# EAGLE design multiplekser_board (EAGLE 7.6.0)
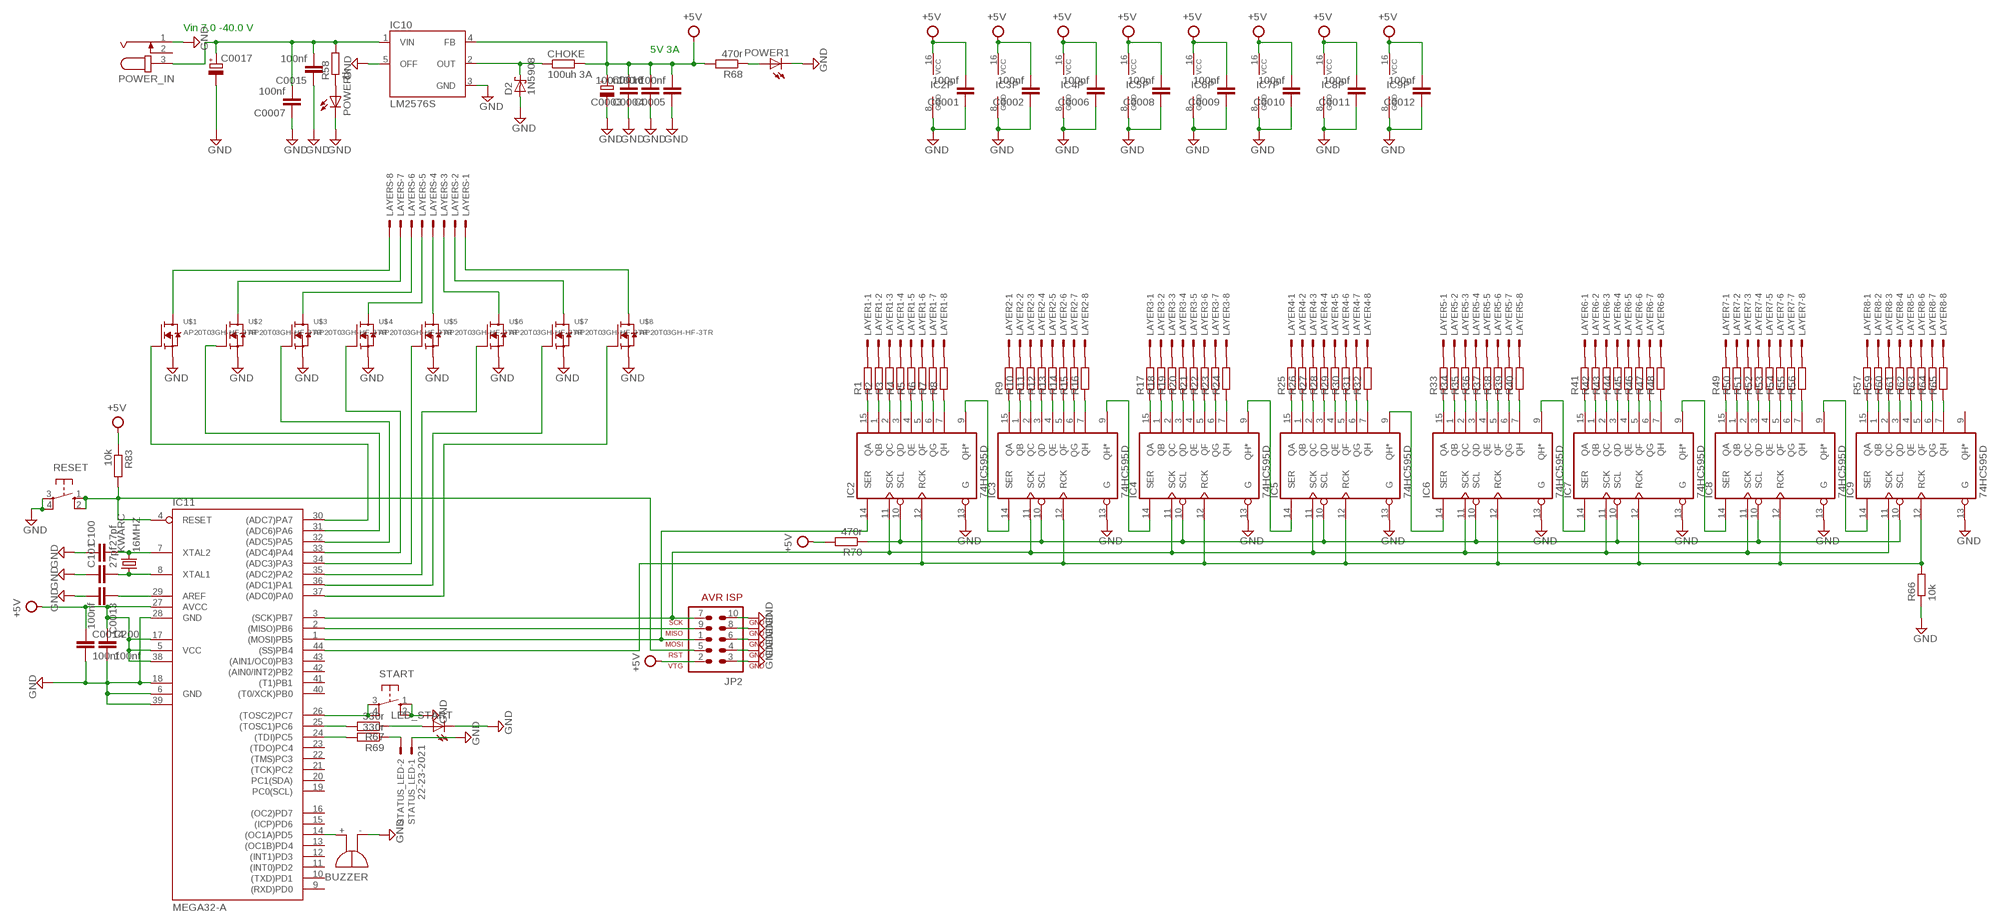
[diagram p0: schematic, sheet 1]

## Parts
BUZZER  F/QMBIII  [F/QMBIII]
C0001  100nf  C-EUC1206  [C1206]
C0002  100nf  C-EUC1206  [C1206]
C0003  100nf  C-EUC1206  [C1206]
C0004  100nf  C-EUC1206  [C1206]
C0005  100nf  C-EUC1206  [C1206]
C0006  100nf  C-EUC1206  [C1206]
C0007  100nf  C-EUC1206  [C1206]
C0008  100nf  C-EUC1206  [C1206]
C0009  100nf  C-EUC1206  [C1206]
C0010  100nf  C-EUC1206  [C1206]
C0011  100nf  C-EUC1206  [C1206]
C0012  100nf  C-EUC1206  [C1206]
C0013  100nf  C-EUC1206  [C1206]
C0014  100nf  C-EUC1206  [C1206]
C0015  100nf  C-EUC1206  [C1206]
C0016  CPOL-EUE10-30  [EB30D]
C0017  CPOL-EUE2.5-6  [E2,5-6]
C100  27pf  C-EUC1206  [C1206]
C101  27pf  C-EUC1206  [C1206]
C200  100nf  C-EUC1206  [C1206]
CHOKE  100uh 3A  R-EU_0207/12  [0207/12]
D2  1N5908  [C4111-15]
IC2  74HC595D  [SO16]
IC3  74HC595D  [SO16]
IC4  74HC595D  [SO16]
IC5  74HC595D  [SO16]
IC6  74HC595D  [SO16]
IC7  74HC595D  [SO16]
IC8  74HC595D  [SO16]
IC9  74HC595D  [SO16]
IC10  LM2576S  [TO263-5]
IC11  MEGA32-A  [TQFP44]
JP2  AVR-ISP-10ML  [ML10]
KWARC  16MHZ  CRYSTALHC49UV  [HC49U-V]
LAYER1  22-23-2081  [22-23-2081]
LAYER2  22-23-2081  [22-23-2081]
LAYER3  22-23-2081  [22-23-2081]
LAYER4  22-23-2081  [22-23-2081]
LAYER5  22-23-2081  [22-23-2081]
LAYER6  22-23-2081  [22-23-2081]
LAYER7  22-23-2081  [22-23-2081]
LAYER8  22-23-2081  [22-23-2081]
LAYERS  22-23-2081  [22-23-2081]
LED_START  LEDCHIPLED_1206  [CHIPLED_1206]
POWER  LEDCHIPLED_1206  [CHIPLED_1206]
POWER1  LEDCHIPLED_1206  [CHIPLED_1206]
POWER_IN  JACK-PLUG1  [SPC4078]
R1  R-EU_M1206  [M1206]
R2  R-EU_M1206  [M1206]
R3  R-EU_M1206  [M1206]
R4  R-EU_M1206  [M1206]
R5  R-EU_M1206  [M1206]
R6  R-EU_M1206  [M1206]
R7  R-EU_M1206  [M1206]
R8  R-EU_M1206  [M1206]
R9  R-EU_M1206  [M1206]
R10  R-EU_M1206  [M1206]
R11  R-EU_M1206  [M1206]
R12  R-EU_M1206  [M1206]
R13  R-EU_M1206  [M1206]
R14  R-EU_M1206  [M1206]
R15  R-EU_M1206  [M1206]
R16  R-EU_M1206  [M1206]
R17  R-EU_M1206  [M1206]
R18  R-EU_M1206  [M1206]
R19  R-EU_M1206  [M1206]
R20  R-EU_M1206  [M1206]
R21  R-EU_M1206  [M1206]
R22  R-EU_M1206  [M1206]
R23  R-EU_M1206  [M1206]
R24  R-EU_M1206  [M1206]
R25  R-EU_M1206  [M1206]
R26  R-EU_M1206  [M1206]
R27  R-EU_M1206  [M1206]
R28  R-EU_M1206  [M1206]
R29  R-EU_M1206  [M1206]
R30  R-EU_M1206  [M1206]
R31  R-EU_M1206  [M1206]
R32  R-EU_M1206  [M1206]
R33  R-EU_M1206  [M1206]
R34  R-EU_M1206  [M1206]
R35  R-EU_M1206  [M1206]
R36  R-EU_M1206  [M1206]
R37  R-EU_M1206  [M1206]
R38  R-EU_M1206  [M1206]
R39  R-EU_M1206  [M1206]
R40  R-EU_M1206  [M1206]
R41  R-EU_M1206  [M1206]
R42  R-EU_M1206  [M1206]
R43  R-EU_M1206  [M1206]
R44  R-EU_M1206  [M1206]
R45  R-EU_M1206  [M1206]
R46  R-EU_M1206  [M1206]
R47  R-EU_M1206  [M1206]
R48  R-EU_M1206  [M1206]
R49  R-EU_M1206  [M1206]
R50  R-EU_M1206  [M1206]
R51  R-EU_M1206  [M1206]
R52  R-EU_M1206  [M1206]
R53  R-EU_M1206  [M1206]
R54  R-EU_M1206  [M1206]
R55  R-EU_M1206  [M1206]
R56  R-EU_M1206  [M1206]
R57  R-EU_M1206  [M1206]
R58  1k  R-EU_R1206  [R1206]
R59  R-EU_M1206  [M1206]
R60  R-EU_M1206  [M1206]
R61  R-EU_M1206  [M1206]
R62  R-EU_M1206  [M1206]
R63  R-EU_M1206  [M1206]
R64  R-EU_M1206  [M1206]
R65  R-EU_M1206  [M1206]
R66  10k  R-EU_M1206  [M1206]
R67  330r  R-EU_M1206  [M1206]
R68  470r  R-EU_R1206  [R1206]
R69  330r  R-EU_M1206  [M1206]
R70  470r  R-EU_M1206  [M1206]
R83  10k  R-EU_R1206  [R1206]
RESET  10-XX  [B3F-10XX]
START  10-XX  [B3F-10XX]
STATUS_LED  22-23-2021  [22-23-2021]
U$1  AP20T03GH-HF-3TR  [TO-252]
U$2  AP20T03GH-HF-3TR  [TO-252]
U$3  AP20T03GH-HF-3TR  [TO-252]
U$4  AP20T03GH-HF-3TR  [TO-252]
U$5  AP20T03GH-HF-3TR  [TO-252]
U$6  AP20T03GH-HF-3TR  [TO-252]
U$7  AP20T03GH-HF-3TR  [TO-252]
U$8  AP20T03GH-HF-3TR  [TO-252]

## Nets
+5V: C0001.2 C0002.2 C0003.2 C0004.2 C0005.2 C0006.2 C0008.2 C0009.2 C0010.2 C0011.2 C0012.2 C0014.1 C0016.+ C200.1 CHOKE.2 IC2.16(VCC) IC3.16(VCC) IC4.16(VCC) IC5.16(VCC) IC6.16(VCC) IC7.16(VCC) IC8.16(VCC) IC9.16(VCC) IC10.4(FB) IC11.5(VCC) IC11.17(VCC1) IC11.27(AVCC) IC11.38(VCC2) JP2.2 R68.2 R70.2 R83.1
GND: BUZZER.-(+) C0001.1 C0002.1 C0003.1 C0004.1 C0005.1 C0006.1 C0007.1 C0008.1 C0009.1 C0010.1 C0011.1 C0012.1 C0013.2 C0014.2 C0015.1 C0016.- C0017.- C100.1 C101.1 C200.2 D2.A IC2.8(GND) IC2.13(G) IC3.8(GND) IC3.13(G) IC4.8(GND) IC4.13(G) IC5.8(GND) IC5.13(G) IC6.8(GND) IC6.13(G) IC7.8(GND) IC7.13(G) IC8.8(GND) IC8.13(G) IC9.8(GND) IC9.13(G) IC10.3(GND) IC10.5(OFF) IC11.6(GND) IC11.18(GND1) IC11.28(GND) IC11.39(GND2) JP2.3 JP2.4 JP2.6 JP2.8 JP2.10 LED_START.C POWER1.C POWER.C POWER_IN.1 R66.1 RESET.3(P) RESET.4(P1) START.1(S) START.2(S1) STATUS_LED.1 U$1.3(S) U$2.3(S) U$3.3(S) U$4.3(S) U$5.3(S) U$6.3(S) U$7.3(S) U$8.3(S)
N$1: IC2.15(QA) R1.1
N$2: IC2.1(QB) R2.1
N$3: IC2.2(QC) R3.1
N$4: IC2.3(QD) R4.1
N$5: IC2.4(QE) R5.1
N$6: IC2.5(QF) R6.1
N$7: IC2.6(QG) R7.1
N$8: IC2.7(QH) R8.1
N$9: IC2.9(QH*) IC3.14(SER)
N$10: IC2.11(SCK) IC3.11(SCK) IC4.11(SCK) IC5.11(SCK) IC6.11(SCK) IC7.11(SCK) IC8.11(SCK) IC9.11(SCK) IC11.3((SCK)PB7) JP2.7
N$11: IC2.12(RCK) IC3.12(RCK) IC4.12(RCK) IC5.12(RCK) IC6.12(RCK) IC7.12(RCK) IC8.12(RCK) IC9.12(RCK) IC11.44((SS)PB4) R66.2
N$12: IC3.15(QA) R9.1
N$13: IC3.1(QB) R10.1
N$14: IC3.2(QC) R11.1
N$15: IC3.3(QD) R12.1
N$16: IC3.4(QE) R13.1
N$17: IC3.5(QF) R14.1
N$18: IC3.6(QG) R15.1
N$19: IC3.7(QH) R16.1
N$20: IC4.15(QA) R17.1
N$21: IC4.1(QB) R18.1
N$22: IC4.2(QC) R19.1
N$23: IC4.3(QD) R20.1
N$24: IC4.4(QE) R21.1
N$25: IC4.5(QF) R22.1
N$26: IC4.6(QG) R23.1
N$27: IC4.7(QH) R24.1
N$28: IC4.9(QH*) IC5.14(SER)
N$29: IC5.15(QA) R25.1
N$30: IC5.1(QB) R26.1
N$31: IC5.2(QC) R27.1
N$32: IC5.3(QD) R28.1
N$33: IC5.4(QE) R29.1
N$34: IC5.5(QF) R30.1
N$35: IC5.6(QG) R31.1
N$36: IC5.7(QH) R32.1
N$37: IC3.9(QH*) IC4.14(SER)
N$38: IC6.3(QD) R36.1
N$39: IC6.4(QE) R37.1
N$40: IC6.5(QF) R38.1
N$41: IC6.6(QG) R39.1
N$42: IC6.7(QH) R40.1
N$43: IC6.9(QH*) IC7.14(SER)
N$44: IC7.15(QA) R41.1
N$45: IC7.1(QB) R42.1
N$46: IC7.2(QC) R43.1
N$47: IC7.3(QD) R44.1
N$48: IC7.4(QE) R45.1
N$49: IC7.5(QF) R46.1
N$50: IC7.6(QG) R47.1
N$51: IC7.7(QH) R48.1
N$52: IC8.15(QA) R49.1
N$53: IC8.1(QB) R50.1
N$54: IC8.2(QC) R51.1
N$55: IC8.3(QD) R52.1
N$56: IC8.4(QE) R53.1
N$57: IC8.5(QF) R54.1
N$58: IC8.6(QG) R55.1
N$59: IC8.7(QH) R56.1
N$60: IC8.9(QH*) IC9.14(SER)
N$61: IC9.15(QA) R57.1
N$62: IC9.1(QB) R59.1
N$63: CHOKE.1 D2.C IC10.2(OUT)
N$64: IC9.2(QC) R60.1
N$65: IC9.3(QD) R61.1
N$66: IC9.4(QE) R62.1
N$67: IC9.5(QF) R63.1
N$68: IC9.6(QG) R64.1
N$69: IC9.7(QH) R65.1
N$70: IC7.9(QH*) IC8.14(SER)
N$71: IC5.9(QH*) IC6.14(SER)
N$72: IC6.15(QA) R33.1
N$73: IC6.1(QB) R34.1
N$74: IC6.2(QC) R35.1
N$75: POWER1.A R68.1
N$76: IC11.4(RESET) JP2.5 R83.2 RESET.1(S) RESET.2(S1)
N$77: C0007.2 C0015.2 C0017.+ IC10.1(VIN) POWER_IN.3 R58.2
N$78: LAYER1.1 R1.2
N$79: LAYER1.2 R2.2
N$80: LAYER1.3 R3.2
N$81: LAYER1.4 R4.2
N$82: LAYER1.5 R5.2
N$83: LAYER1.6 R6.2
N$84: LAYER1.7 R7.2
N$85: LAYER1.8 R8.2
N$86: LAYER2.1 R9.2
N$87: LAYER2.2 R10.2
N$88: LAYER2.3 R11.2
N$89: LAYER2.4 R12.2
N$90: LAYER2.5 R13.2
N$91: LAYER2.6 R14.2
N$92: LAYER2.7 R15.2
N$93: LAYER2.8 R16.2
N$94: LAYER3.1 R17.2
N$95: LAYER3.2 R18.2
N$96: LAYER3.3 R19.2
N$97: LAYER3.4 R20.2
N$98: LAYER3.5 R21.2
N$99: LAYER3.6 R22.2
N$100: LAYER3.7 R23.2
N$101: LAYER3.8 R24.2
N$102: LAYER4.1 R25.2
N$103: LAYER4.2 R26.2
N$104: LAYER4.3 R27.2
N$105: LAYER4.4 R28.2
N$106: LAYER4.5 R29.2
N$107: LAYER4.6 R30.2
N$108: LAYER4.7 R31.2
N$109: LAYER4.8 R32.2
N$110: LAYER5.1 R33.2
N$111: LAYER5.2 R34.2
N$112: LAYER5.3 R35.2
N$113: LAYER5.4 R36.2
N$114: LAYER5.5 R37.2
N$115: LAYER5.6 R38.2
N$116: LAYER5.7 R39.2
N$117: LAYER5.8 R40.2
N$118: LAYER6.1 R41.2
N$119: IC11.2((MISO)PB6) JP2.9
N$120: LAYER6.2 R42.2
N$121: LAYER6.3 R43.2
N$122: LAYER6.4 R44.2
N$123: LAYER6.5 R45.2
N$124: LAYER6.6 R46.2
N$125: LAYER6.7 R47.2
N$126: LAYER6.8 R48.2
N$127: LAYER7.1 R49.2
N$128: LAYER7.2 R50.2
N$129: LAYER7.3 R51.2
N$130: LAYER7.4 R52.2
N$131: LAYER7.5 R53.2
N$132: LAYER7.6 R54.2
N$133: LAYER7.7 R55.2
N$134: LAYER7.8 R56.2
N$135: LAYER8.1 R57.2
N$136: LAYER8.2 R59.2
N$137: LAYER8.3 R60.2
N$138: LAYER8.4 R61.2
N$139: LAYER8.5 R62.2
N$140: LAYER8.6 R63.2
N$141: LAYER8.7 R64.2
N$142: LAYER8.8 R65.2
N$143: LAYERS.8 U$1.2(D)
N$144: LAYERS.7 U$2.2(D)
N$145: LAYERS.6 U$3.2(D)
N$146: LAYERS.5 U$4.2(D)
N$147: IC2.14(SER) IC11.1((MOSI)PB5) JP2.1
N$148: LAYERS.4 U$5.2(D)
N$149: LAYERS.3 U$6.2(D)
N$150: LAYERS.2 U$7.2(D)
N$151: LAYERS.1 U$8.2(D)
N$152: IC11.30((ADC7)PA7) U$1.1(G)
N$153: IC11.31((ADC6)PA6) U$2.1(G)
N$154: IC11.32((ADC5)PA5) U$3.1(G)
N$155: IC11.33((ADC4)PA4) U$4.1(G)
N$156: IC11.34((ADC3)PA3) U$5.1(G)
N$157: IC11.35((ADC2)PA2) U$6.1(G)
N$158: IC11.36((ADC1)PA1) U$7.1(G)
N$159: IC11.37((ADC0)PA0) U$8.1(G)
N$160: BUZZER.+(-) IC11.14((OC1A)PD5)
N$161: IC11.26((TOSC2)PC7) START.3(P) START.4(P1)
N$162: IC11.25((TOSC1)PC6) R67.2
N$163: LED_START.A R67.1
N$164: IC11.24((TDI)PC5) R69.2
N$165: R69.1 STATUS_LED.2
N$166: IC2.10(SCL) IC3.10(SCL) IC4.10(SCL) IC5.10(SCL) IC6.10(SCL) IC7.10(SCL) IC8.10(SCL) IC9.10(SCL) R70.1
N$182: C0013.1 IC11.29(AREF)
N$186: POWER.A R58.1
N$187: C101.2 IC11.8(XTAL1) KWARC.1
N$188: C100.2 IC11.7(XTAL2) KWARC.2
Unconnected: IC9.9(QH*) IC11.9((RXD)PD0) IC11.10((TXD)PD1) IC11.11((INT0)PD2) IC11.12((INT1)PD3) IC11.13((OC1B)PD4) IC11.15((ICP)PD6) IC11.16((OC2)PD7) IC11.19(PC0(SCL)) IC11.20(PC1(SDA)) IC11.21((TCK)PC2) IC11.22((TMS)PC3) IC11.23((TDO)PC4) IC11.40((T0/XCK)PB0) IC11.41((T1)PB1) IC11.42((AIN0/INT2)PB2) IC11.43((AIN1/OC0)PB3) POWER_IN.2

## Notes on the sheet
- Vin 7.0 -40.0 V
- 5V 3A

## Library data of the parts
BUZZER = buzzer:F/QMBIII: BUZZER; OC_FARNELL: unknown; OC_NEWARK: unknown
C0001-C0009 C0010-C0015 C100 C101 C200 = rcl:C-EU: CAPACITOR, European symbol
C0016 = rcl:CPOL-EU: POLARIZED CAPACITOR, European symbol
C0017 = resistor:CPOL-EU: POLARIZED CAPACITOR, European symbol
CHOKE = rcl:R-EU_: RESISTOR, European symbol
D2 = diode:1N5908: DIODE
IC2-IC9 = 74xx-eu:74*595: 8-bit SHIFT REGISTER, output latch
IC10 = v-reg-3:LM2576: National Semiconductor 3.0A "Simple Switcher"(c) 52kHz, Vout 1.23-37V (HV: 57V), Vin 40V (HV: 60V), 50µA standby current
IC11 = atmel:MEGA32: MICROCONTROLLER 32 Kbytes FLASH 2 Kbytes SRAM 1 Kbytes EEPROM USART 8-channel 10 bit ADC Source: www.atmel.com .. doc2503.pdf; MPN: ATMEGA32-16AU; OC_FARNELL: 9171274; OC_NEWARK: 69K6677
JP2 = atmel-1:AVR-ISP-10: AVR ISP-10 Serial Programming Header
KWARC = SparkFun:CRYSTAL: Crystals
LAYER1-LAYER8 LAYERS = con-molex:22-23-2081: .100" (2.54mm) Center Header - 8 Pin; MF: MOLEX; MPN: 22-23-2081; OC_FARNELL: 1756826; OC_NEWARK: 01C7592
LED_START POWER POWER1 = led:LED: LED
POWER_IN = tango:JACK-PLUG: DC POWER JACK Power Jack, DC, Right Angle, Through Hole, Rated 5A at 16VDC, PC Terminals Distributor: Farnell (www.Farnell.de) Drawing: 84N1161.pdf / 84N1162.pdf Manufacturer: SPC Technology (www.spctechnology.com) Type: SPC4077 / SPC 4078
R1-R57 R59-R67 R69 R70 = resistor:R-EU_: RESISTOR, European symbol
R58 R68 R83 = rcl-2:R-EU_: RESISTOR, European symbol
RESET START = switch-omron:10-XX: OMRON SWITCH; MPN: B3F-1000; OC_FARNELL: 176432; OC_NEWARK: 36M3542
STATUS_LED = con-molex:22-23-2021: .100" (2.54mm) Center Header - 2 Pin; MF: MOLEX; MPN: 22-23-2021; OC_FARNELL: 1462926; OC_NEWARK: 25C3832
U$1-U$8 = APEC:AP20T03GH-HF-3TR

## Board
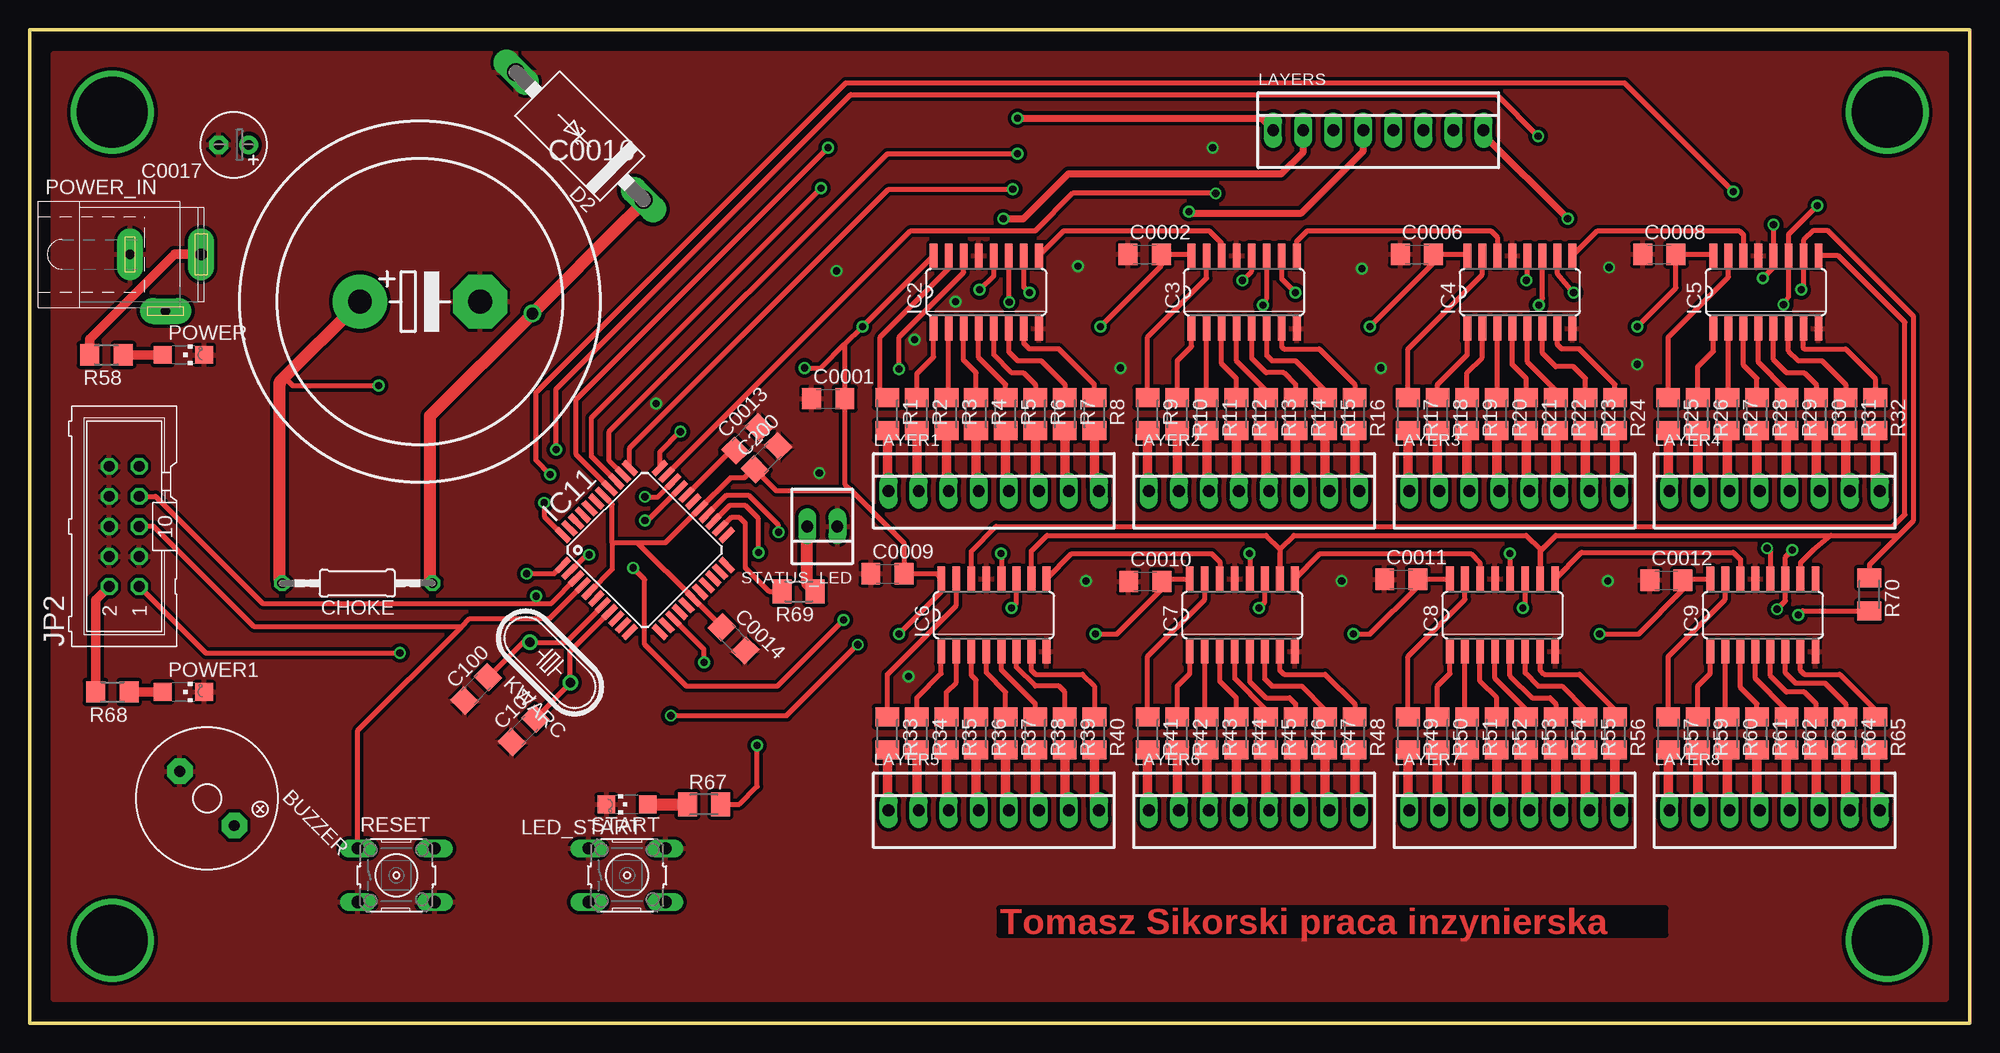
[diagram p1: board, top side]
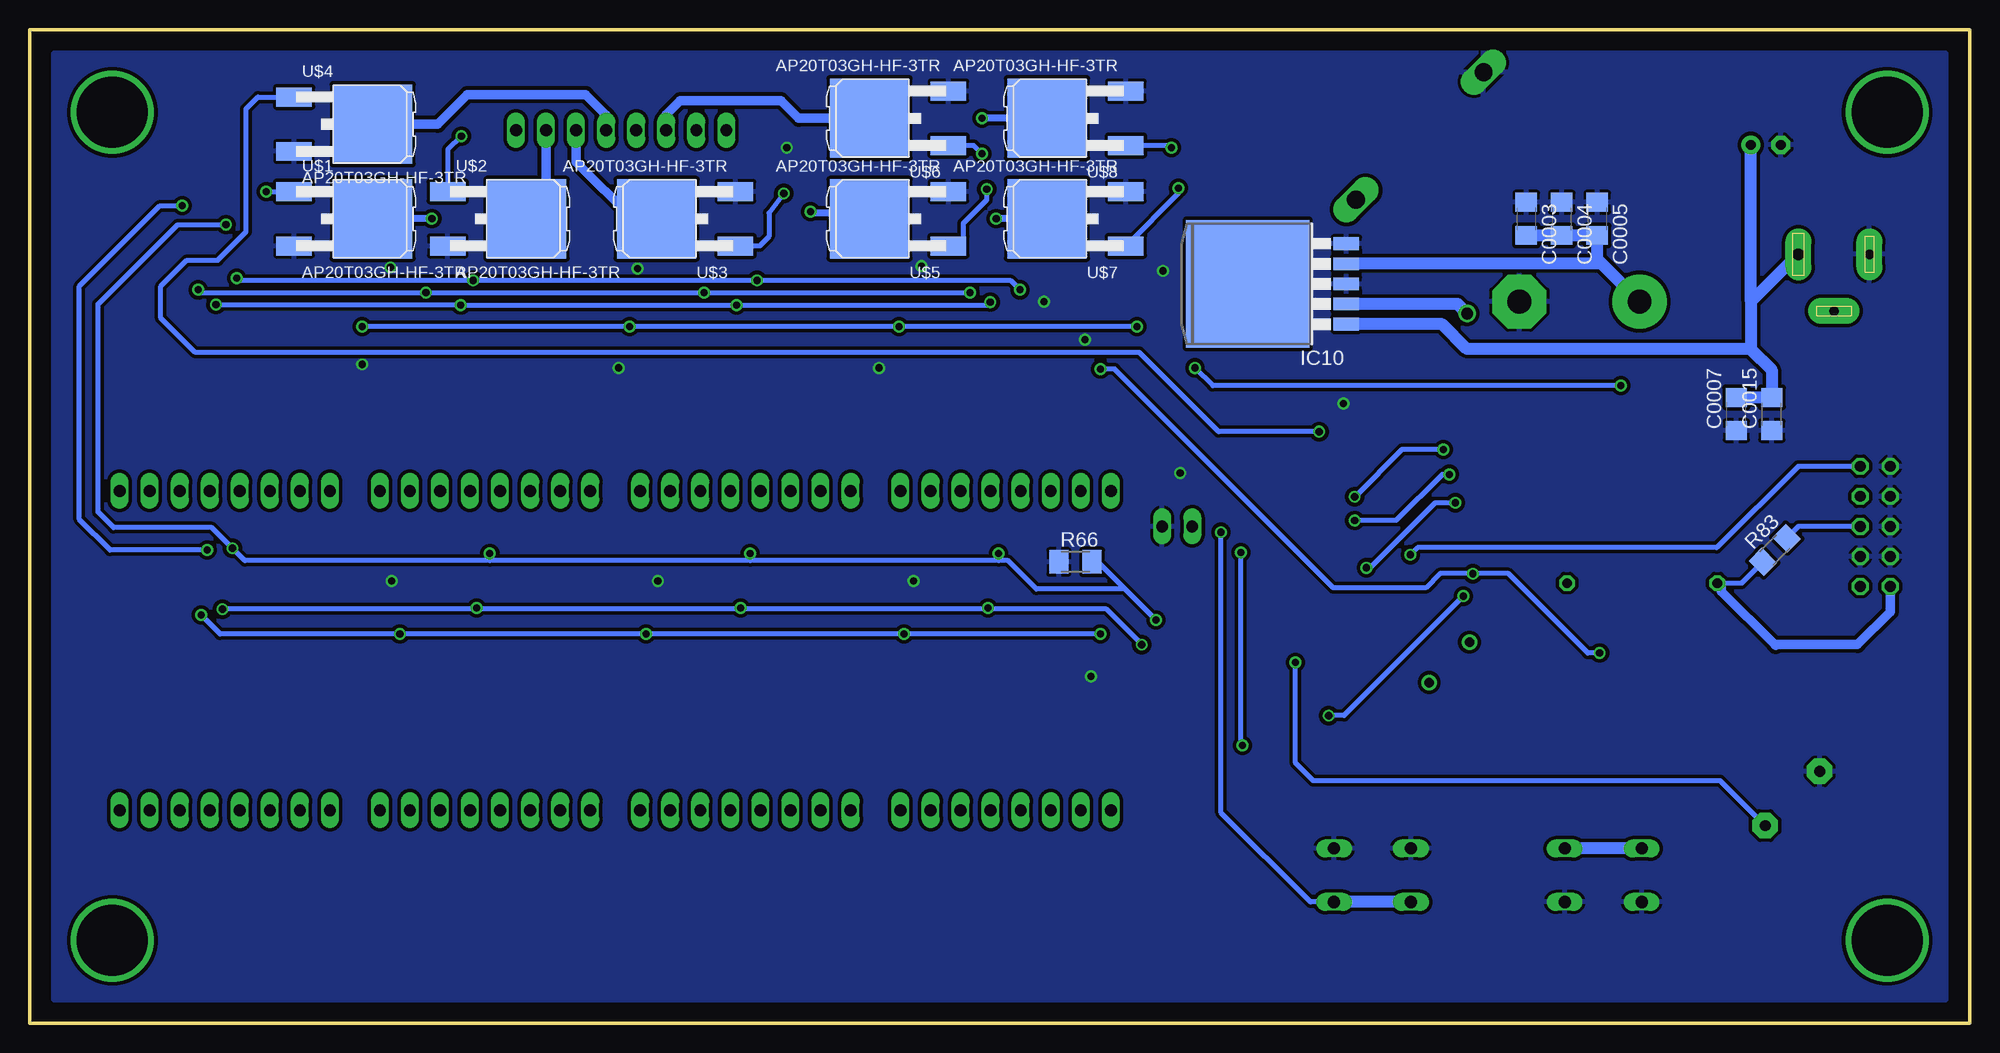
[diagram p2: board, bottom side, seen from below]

Size 164 x 84 mm. Coordinates in mm from the lower left corner, seen from the top.
Outline: 0,0 164,0 164,84 0,84 0,0
Copper layers (1*16): Top 0.035mm / dielectric 1.5mm / Bottom 0.035mm
Design rules "default": minimum track width 10mil, minimum drill 24mil, track to track 8mil, track to pad 8mil, pad to pad 8mil, via to via 8mil, smd to smd 8mil, copper to edge 40mil, drill to drill 8mil, minimum pad ring 10mil, minimum via ring 8mil, stop-mask expansion 4mil, vias tented up to drill 0mil, thermal gap 10mil

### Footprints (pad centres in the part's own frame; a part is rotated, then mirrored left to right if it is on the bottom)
F/QMBIII = drill 0.914 pad 2.159 octagon: + 3.251,0; - -3.251,0
C1206 = smd 1.6 x 1.8: 1 -1.4,0; 2 1.4,0
EB30D = drill 2.007 pad 4.597: + -5.08,0 | drill 2.007 pad 4.597 octagon: - 5.08,0
E2,5-6 = drill 0.813 pad 1.6: + -1.27,0 | drill 0.813 pad 1.6 octagon: - 1.27,0
0207/12 = drill 0.813 octagon: 1 -6.35,0; 2 6.35,0
C4111-15 = drill 1.499 long: A 7.62,0; C -7.62,0
SO16 = smd 0.66 x 2.032: 1 -4.445,-3.073; 2 -3.175,-3.073; 3 -1.905,-3.073; 4 -0.635,-3.073; 5 0.635,-3.073; 6 1.905,-3.073; 7 3.175,-3.073; 8 4.445,-3.073; 9 4.445,3.073; 10 3.175,3.073; 11 1.905,3.073; 12 0.635,3.073; 13 -0.635,3.073; 14 -1.905,3.073; 15 -3.175,3.073; 16 -4.445,3.073
TO263-5 = smd 1.067 x 2.159: 1 -3.404,-5.791; 2 -1.702,-5.791; 3 0,-5.791; 4 1.702,-5.791; 5 3.404,-5.791 | smd 10.8 x 10.41: 6 0,2.54
TQFP44 = smd 1.5 x 0.5: 1 -5.8,4; 2 -5.8,3.2; 3 -5.8,2.4; 4 -5.8,1.6; 5 -5.8,0.8; 6 -5.8,0; 7 -5.8,-0.8; 8 -5.8,-1.6; 9 -5.8,-2.4; 10 -5.8,-3.2; 11 -5.8,-4; 23 5.8,-4; 24 5.8,-3.2; 25 5.8,-2.4; 26 5.8,-1.6; 27 5.8,-0.8; 28 5.8,0; 29 5.8,0.8; 30 5.8,1.6; 31 5.8,2.4; 32 5.8,3.2; 33 5.8,4 | smd 0.5 x 1.5: 12 -4,-5.8; 13 -3.2,-5.8; 14 -2.4,-5.8; 15 -1.6,-5.8; 16 -0.8,-5.8; 17 0,-5.8; 18 0.8,-5.8; 19 1.6,-5.8; 20 2.4,-5.8; 21 3.2,-5.8; 22 4,-5.8; 34 4,5.8; 35 3.2,5.8; 36 2.4,5.8; 37 1.6,5.8; 38 0.8,5.8; 39 0,5.8; 40 -0.8,5.8; 41 -1.6,5.8; 42 -2.4,5.8; 43 -3.2,5.8; 44 -4,5.8
ML10 = drill 0.914 octagon: 1 -5.08,-1.27; 2 -5.08,1.27; 3 -2.54,-1.27; 4 -2.54,1.27; 5 0,-1.27; 6 0,1.27; 7 2.54,-1.27; 8 2.54,1.27; 9 5.08,-1.27; 10 5.08,1.27
HC49U-V = drill 0.813: 1 -2.413,0; 2 2.413,0
22-23-2081 = drill 1 long: 1 -8.89,0; 2 -6.35,0; 3 -3.81,0; 4 -1.27,0; 5 1.27,0; 6 3.81,0; 7 6.35,0; 8 8.89,0
CHIPLED_1206 = smd 1.5 x 1.5: A 0,-1.75; C 0,1.75
SPC4078 = drill 0.8 pad 2.184 long: 1 -3,0; 2 0,-4.8 | drill 1 pad 2.184 long: 3 3,0
M1206 = smd 1.6 x 2: 1 -1.4,0; 2 1.4,0
R1206 = smd 1.6 x 1.803: 1 -1.422,0; 2 1.422,0
B3F-10XX = drill 1.016 long: 1 -3.251,2.261; 2 3.251,2.261; 3 -3.251,-2.261; 4 3.251,-2.261
22-23-2021 = drill 1 long: 1 -1.27,0; 2 1.27,0
TO-252 = smd 1.6 x 3: 1 -2.3,-6.65; 3 2.3,-6.65 | smd 6.7 x 6.7: 2 0,0

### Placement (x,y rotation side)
BUZZER  15,19 315 top
C0001  67.5,52.8 0 top
C0002  94.25,65 0 top
C0003  37.5,68 270 bottom
C0004  34.5,68 270 bottom
C0005  31.5,68 270 bottom
C0006  117.25,65 0 top
C0007  19.75,51.5 90 bottom
C0008  137.75,65 0 top
C0009  72.5,38 0 top
C0010  94.3,37.35 0 top
C0011  115.93,37.52 0 top
C0012  138.35,37.45 0 top
C0013  60.65,49.4 45 top
C0014  59.5,32.5 315 top
C0015  16.75,51.5 90 bottom
C0016  33,61 0 top
C0017  17.25,74.25 180 top
C100  37.75,28.25 45 top
C101  41.75,24.75 45 top
C200  62.3,47.8 45 top
CHOKE  27.7,37.2 180 top
D2  46.5,75 135 top
IC2  80.86,61.81 0 top
IC3  102.66,61.81 0 top
IC4  125.96,61.81 0 top
IC5  146.76,61.81 0 top
IC6  81.5,34.5 0 top
IC7  102.5,34.5 0 top
IC8  124.5,34.5 0 top
IC9  146.5,34.5 0 top
IC10  58.5,62.5 90 bottom
IC11  52,40 45 top
JP2  8,42 90 top
KWARC  44,30.5 135 top
LAYER1  81.5,45 0 top
LAYER2  103.5,45 0 top
LAYER3  125.5,45 0 top
LAYER4  147.5,45 0 top
LAYER5  81.5,18 0 top
LAYER6  103.5,18 0 top
LAYER7  125.5,18 0 top
LAYER8  147.5,18 0 top
LAYERS  114,75.5 0 top
LED_START  50.5,18.5 90 top
POWER  13,56.5 270 top
POWER1  13,28 270 top
POWER_IN  11.5,65 0 top
R1  72.5,51.5 270 top
R2  75,51.5 270 top
R3  77.5,51.5 270 top
R4  80,51.5 270 top
R5  82.5,51.5 270 top
R6  85,51.5 270 top
R7  87.5,51.5 270 top
R8  90,51.5 270 top
R9  94.5,51.5 270 top
R10  97,51.5 270 top
R11  99.5,51.5 270 top
R12  102,51.5 270 top
R13  104.5,51.5 270 top
R14  107,51.5 270 top
R15  109.5,51.5 270 top
R16  112,51.5 270 top
R17  116.5,51.5 270 top
R18  119,51.5 270 top
R19  121.5,51.5 270 top
R20  124,51.5 270 top
R21  126.5,51.5 270 top
R22  129,51.5 270 top
R23  131.5,51.5 270 top
R24  134,51.5 270 top
R25  138.5,51.5 270 top
R26  141,51.5 270 top
R27  143.5,51.5 270 top
R28  146,51.5 270 top
R29  148.5,51.5 270 top
R30  151,51.5 270 top
R31  153.5,51.5 270 top
R32  156,51.5 270 top
R33  72.5,24.5 270 top
R34  75,24.5 270 top
R35  77.5,24.5 270 top
R36  80,24.5 270 top
R37  82.5,24.5 270 top
R38  85,24.5 270 top
R39  87.5,24.5 270 top
R40  90,24.5 270 top
R41  94.5,24.5 270 top
R42  97,24.5 270 top
R43  99.5,24.5 270 top
R44  102,24.5 270 top
R45  104.5,24.5 270 top
R46  107,24.5 270 top
R47  109.5,24.5 270 top
R48  112,24.5 270 top
R49  116.5,24.5 270 top
R50  119,24.5 270 top
R51  121.5,24.5 270 top
R52  124,24.5 270 top
R53  126.5,24.5 270 top
R54  129,24.5 270 top
R55  131.5,24.5 270 top
R56  134,24.5 270 top
R57  138.5,24.5 270 top
R58  6.5,56.5 180 top
R59  141,24.5 270 top
R60  143.5,24.5 270 top
R61  146,24.5 270 top
R62  148.5,24.5 270 top
R63  151,24.5 270 top
R64  153.5,24.5 270 top
R65  156,24.5 270 top
R66  75.6,39 0 bottom
R67  57,18.5 0 top
R68  7,28 180 top
R69  65,36.5 180 top
R70  155.5,36.25 270 top
R83  16.5,40 45 bottom
RESET  31,12.5 0 top
START  50.5,12.5 0 top
STATUS_LED  67,42 180 top
U$1  135,68 270 bottom
U$2  122,68 270 bottom
U$3  111,68 90 bottom
U$4  135,76 270 bottom
U$5  93,68 90 bottom
U$6  93,76.5 90 bottom
U$7  78,68 90 bottom
U$8  78,76.5 90 bottom

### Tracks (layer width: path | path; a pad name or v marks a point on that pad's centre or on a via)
+5V  (via drill 0.6)
  Top 0.406: 149.68,34.67 v149.5,34.5 149.85,34.85 R70.2 | IC3.16 98.1,65 C0002.2 95.65,64.05 v90.5,58.9 | IC4.16 121.4,65 C0006.2 118.65,64.25 v113.3,58.9 | 21.15,54 21.65,54.5 22.25,53.9 v29.5,53.9 | IC11.5 49.25,38.38 49.25,40.6 | 49.25,40.6 49.25,43.88 IC11.38 | C0014.1 IC11.17 51.4,40.6 | 51.4,40.6 49.25,40.6 | 51.4,40.6 53.73,40.6 IC11.27 59.23,46.1 60.4,46.1 60.81,46.51 C200.1 63.12,45 69.5,45 | IC7.16 95.92,37.57 C0010.2 95.7,36.7 91.9,32.9 v90.1,32.9 | IC8.16 117.38,37.57 C0011.2 117.33,36.93 113.3,32.9 v111.9,32.9 | IC9.16 139.87,37.57 C0012.2 139.75,36.65 136,32.9 v132.7,32.9 | 75.92,64.41 76.42,64.41 IC2.16 76.38,64.88 v70.4,58.9 68.9,57.4 | 68.9,57.4 C0001.2 68.9,45.6 69.5,45 | v65.5,55.4 66.9,55.4 68.9,57.4 | v135.9,58.9 139.15,62.15 C0008.2 142.2,65 IC5.16 | 69.5,45 73.9,40.6 C0009.2 76.63,38 IC6.16 77.06,36.45 v73.5,32.9 73.4,32.9
  Top 0.813: R68.2 5.58,35.77 JP2.2
  Top 1.016: C0016.+ 21.15,54.23 21.15,54 21.15,37.4 CHOKE.2
  Bottom 0.406: R83.1 19.3,37.2 CHOKE.2 | v29.5,53.9 64,53.9 v65.5,55.4 | v70.4,58.9 v90.5,58.9 v113.3,58.9 v135.9,58.9 | v149.5,34.5 147.9,32.9 v132.7,32.9 v111.9,32.9 v90.1,32.9 v73.5,32.9
  Bottom 0.813: JP2.2 6.73,34.77 9.5,32 16.5,32 | 16.5,32 21,36.5 21,36.85 CHOKE.2 | 16.5,32 16.42,31.92
  Bottom 1.016: 31.12,64.2 IC10.4 | C0016.+ 31.12,64.2 | C0003.2 C0004.2 C0005.2 31.5,64.58 31.12,64.2
GND  (via drill 0.6)
  other vias: 52.95,52.4 68.2,63.6 135.9,55.7 114.2,55.4 92.2,55.4 100,74 66.75,46.5 74.8,57.8 88.6,64 112.6,63.8 133.5,63.9 133.4,37.4 110.9,37.4 89.3,37.4 74.3,29.3 78.25,61
  pour Bottom (isolate 0.305): 2,82 162,82 162,2 2,2
  pour Top (isolate 0.305): 2,82 162,82 162,2 2,2
N$1
  Top 0.406: IC2.15 77.69,63.78 71.9,58 71.9,53.5 R1.1
N$2
  Top 0.406: IC2.1 76.42,56.31 75,54.9 R2.1
N$3
  Top 0.406: IC2.2 77.69,53.09 arc-90 R3.1
N$4
  Top 0.406: IC2.3 78.95,56.05 80,55 R4.1
N$5
  Top 0.406: IC2.4 80.22,56.27 82.5,54 R5.1
N$6
  Top 0.406: IC2.5 81.5,56.51 83,55 84,55 85,54 R6.1
N$7
  Top 0.406: IC2.6 82.77,56.73 83.5,56 85.5,56 87.5,54 R7.1
N$8
  Top 0.406: IC2.7 84.03,57.47 84.5,57 87,57 90,54 R8.1 90,52.5
N$9
  Top 0.406: IC2.9 87.42,67 99.7,67 100.7,66 100.7,64.94 IC3.14
N$10  (via drill 0.6)
  Top 0.406: v149,40 148.41,39.41 IC9.11 148.41,35.7 v147.7,35 | v151.1,69.1 148.66,66.67 IC5.11 148.66,61.41 v148.25,60.75 | IC11.3 44.11,35.5 42.8,35.5 | 9.46,44.54 JP2.7 10.66,44.54 19.7,35.5 42.8,35.5 | 42.8,35.5 v42.8,36.1 | v70,32 64,26 v54.2,26 | IC4.11 127.86,61.27 v127.55,60.7 | IC3.11 104.56,61.27 v104.25,60.7 | IC2.11 82.77,61.23 v82.8,60.95 | IC8.11 126.41,35.3 v126.2,35.1 | IC7.11 104.41,35.6 v103.9,35.1 | IC6.11 83.41,35.51 v83,35.1
  Bottom 0.406: v42.8,36.1 52.9,26 v54.2,26 | v149,40 157.2,40 159.8,42.6 159.8,62.3 153,69.1 v151.1,69.1 | v70,32 73,35 82.8,35 | 126.1,35 v147.7,35 | 126.1,35 v126.2,35.1 | 82.8,35 103.8,35 | 103.8,35 126.1,35 | 103.8,35 v103.9,35.1 | v83,35.1 82.9,35.1 82.8,35 | v148.25,60.75 127.85,60.75 v127.55,60.7 v104.25,60.7 83.05,60.7 v82.8,60.95
N$11  (via drill 0.6)
  Top 0.406: v147.4,67.5 147.4,66.89 IC5.12 147.4,63.9 v146.5,63 | v51,38.5 52,37.5 52,32 55.5,28.5 63.2,28.5 v68.8,34.1 | v43.5,44 43.5,42.84 IC11.44 | IC2.12 81.5,63.2 v80.3,62 | IC3.12 103.3,63.59 v102.5,62.8 | IC4.12 126.59,62.9 v126.5,62.8 | IC6.12 82.14,39.66 v82.1,39.7 | IC7.12 103.14,39.66 v103.1,39.7 | IC8.12 125.14,39.66 v125.1,39.7 | IC9.12 147.13,39.87 v146.85,40.15
  Bottom 0.406: v147.4,67.5 151.5,67.5 158.2,60.8 158.2,43.2 156.9,41.9 148.6,41.9 v146.85,40.15 145.8,39.1 125.1,39.1 | v43.5,44 45.2,44 50.7,38.5 v51,38.5 | v80.3,62 81.1,62.8 v102.5,62.8 v126.5,62.8 146.5,62.8 v146.5,63 | 82.1,39.1 81.3,39.1 78.9,36.7 71.4,36.7 | 82.1,39.1 103.1,39.1 | 103.1,39.1 125.1,39.1 | 82.1,39.1 v82.1,39.7 | 103.1,39.1 v103.1,39.7 | 125.1,39.1 v125.1,39.7 | v68.8,34.1 71.4,36.7 | R66.2 73.7,39 71.4,36.7
N$12
  Top 0.406: IC3.15 99.48,62.98 94.5,58 R9.1
N$13
  Top 0.406: IC3.1 98.22,57.22 97,56 R10.1
N$14
  Top 0.406: IC3.2 99.48,52.91 R11.1
N$15
  Top 0.406: IC3.3 100.75,55.74 102,54.5 R12.1
N$16
  Top 0.406: IC3.4 102.03,55.98 104.5,53.5 R13.1
N$17
  Top 0.406: IC3.5 103.3,56.2 104.5,55 106,55 107,54 R14.1
N$18
  Top 0.406: IC3.6 104.56,56.44 105,56 107,56 109.5,53.5 R15.1
N$19
  Top 0.406: IC3.7 105.83,57.16 106,57 109,57 112,54 R16.1
N$20
  Top 0.406: IC4.15 122.78,63.28 116.5,57 R17.1
N$21
  Top 0.406: IC4.1 121.52,56.52 119,54 R18.1
N$22
  Top 0.406: IC4.2 122.78,56.28 121.5,55 R19.1
N$23
  Top 0.406: IC4.3 124.06,52.9 R20.1
N$24
  Top 0.406: IC4.4 125.33,55.67 126.5,54.5 R21.1
N$25
  Top 0.254: R22.1 129,52.8
  Top 0.406: IC4.5 126.59,55.91 129,53.5 R22.1
N$26
  Top 0.406: IC4.6 127.86,56.63 129,55.5 130.5,55.5 131.5,54.5 R23.1
N$27
  Top 0.406: IC4.7 129.13,57.37 129.5,57 131,57 134,54 R24.1
N$28
  Top 0.406: IC5.14 144.85,66.64 144.5,67 132.52,67 IC4.9
N$29
  Top 0.406: IC5.15 143.59,63.09 138.5,58 R25.1
N$30
  Top 0.406: IC5.1 142.31,56.81 141,55.5 R26.1
N$31
  Top 0.406: IC5.2 143.59,52.9 R27.1
N$32
  Top 0.406: IC5.3 144.85,55.65 146,54.5 R28.1
N$33
  Top 0.406: IC5.4 146.12,55.88 148.5,53.5 R29.1
N$34
  Top 0.406: IC5.5 147.4,56.1 148.5,55 150,55 151,54 R30.1
N$35
  Top 0.406: IC5.6 148.66,56.84 149.5,56 151.5,56 153.5,54 R31.1
N$36
  Top 0.406: IC5.7 149.94,57.06 150,57 153.5,57 156,54.5 R32.1
N$37
  Top 0.406: IC4.14 124.06,66.44 123.5,67 108,67 107.11,66.11 IC3.9
N$38
  Top 0.406: IC6.3 79.59,29.41 80,29 R36.1
N$39
  Top 0.406: IC6.4 80.86,29.64 82.5,28 R37.1
N$40
  Top 0.406: IC6.5 82.14,29.86 85,27 R38.1
N$41
  Top 0.406: IC6.6 83.41,30.09 85,28.5 87,28.5 87.5,28 R39.1
N$42
  Top 0.406: IC6.7 84.67,29.82 85,29.5 89,29.5 90,28.5 R40.1
N$43
  Top 0.406: IC7.14 100.59,39.01 99.9,39.7 88.07,39.7 IC6.9
N$44
  Top 0.406: IC7.15 99.33,35.83 94.5,31 R41.1
N$45
  Top 0.406: IC7.1 98.06,29.55 97,28.5 R42.1
N$46
  Top 0.406: 99.33,26.07 R43.1 99.33,25.9 IC7.2
N$47
  Top 0.406: IC7.3 100.59,28.91 102,27.5 R44.1
N$48
  Top 0.406: IC7.4 101.86,29.14 104.5,26.5 R45.1
N$49
  Top 0.406: IC7.5 103.14,28.86 104.5,27.5 106.5,27.5 107,27 R46.1
N$50
  Top 0.406: IC7.6 104.41,29.09 105,28.5 107.5,28.5 109.5,26.5 R47.1
N$51
  Top 0.406: IC7.7 105.67,29.82 106,29.5 109.5,29.5 112,27 R48.1
N$52
  Top 0.406: IC8.15 121.33,35.83 116.5,31 R49.1
N$53
  Top 0.406: IC8.1 120.06,29.55 119,28.5 R50.1
N$54
  Top 0.406: IC8.2 121.33,26.07 R51.1
N$55
  Top 0.406: IC8.3 122.59,28.91 124,27.5 R52.1
N$56
  Top 0.406: IC8.4 123.86,29.14 126.5,26.5 R53.1 126.5,25.5
N$57
  Top 0.406: IC8.5 125.14,29.36 127,27.5 128.5,27.5 129,27 R54.1
N$58
  Top 0.406: IC8.6 126.41,29.59 127.5,28.5 129.5,28.5 131.5,26.5 R55.1
N$59
  Top 0.406: IC8.7 127.67,29.82 128,29.5 131,29.5 134,26.5 R56.1
N$60
  Top 0.406: IC9.14 144.59,39.2 144,39.8 131.17,39.8 IC8.9
N$61
  Top 0.406: IC9.15 143.32,35.83 138.5,31 R57.1
N$62
  Top 0.406: IC9.1 142.06,29.55 141,28.5 R59.1 141.5,25.9
N$63  (via drill 1)
  Top 1.016: CHOKE.1 33.85,37.4 33.85,51.35 v42.5,60 50.5,68 51.09,68.59 51.89,69.39 D2.C
  Bottom 1.016: IC10.2 43.3,60.8 v42.5,60
N$64
  Top 0.406: IC9.2 143.32,26.07 R60.1
N$65
  Top 0.406: IC9.3 144.59,28.41 146,27 R61.1
N$66
  Top 0.406: IC9.4 145.87,29.14 148.5,26.5 R62.1
N$67
  Top 0.406: IC9.5 147.13,29.36 148.5,28 150,28 151,27 R63.1
N$68
  Top 0.406: R64.1 153.5,27 151.75,28.75 149.25,28.75 148.41,29.59 IC9.6
N$69
  Top 0.406: IC9.7 149.68,29.82 150,29.5 153,29.5 156,26.5 R65.1
N$70
  Top 0.406: IC8.14 122.59,38.91 121.8,39.7 109.07,39.7 IC7.9
N$71
  Top 0.406: IC6.14 79.59,39.9 81.7,42 157.5,42 158.5,43 158.5,59.25 152.87,64.88 IC5.9
N$72
  Top 0.406: IC6.15 78.33,35.33 72.5,29.5 R33.1
N$73
  Top 0.406: IC6.1 77.06,29.55 75,27.5 R34.1
N$74
  Top 0.406: IC6.2 78.33,28.82 77.5,28 R35.1
N$75
  Top 0.813: R68.1 POWER1.A
N$76
  Top 0.406: JP2.5 10.5,42 19,33.5 36.5,33.5 | RESET.1 27.75,24.75 36.5,33.5 | IC11.4 43.94,34.2 37.2,34.2 36.5,33.5
  Bottom 0.406: R83.2 14.5,42 JP2.5
  Bottom 1.016: RESET.1 RESET.2
N$77
  Top 0.813: R58.2 5.08,57.83 12.25,65 POWER_IN.3
  Bottom 1.016: IC10.1 44.6,59.1 42.5,57 18.5,57 | 18.5,57 16.75,55.25 C0015.2 C0007.2 | POWER_IN.3 18.5,61 | 18.5,61 18.5,60.75 18.5,57 | C0017.+ 18.5,74.23 18.5,61
N$78
  Top 0.813: R1.2 72.5,45.11 LAYER1.1
N$79
  Top 0.813: R2.2 75,45.15 LAYER1.2
N$80
  Top 0.813: R3.2 77.5,45.19 LAYER1.3
N$81
  Top 0.813: R4.2 80,45.23 LAYER1.4
N$82
  Top 0.813: R5.2 82.5,45.27 LAYER1.5
N$83
  Top 0.813: R6.2 85,45.31 LAYER1.6
N$84
  Top 0.813: R7.2 87.5,45.35 LAYER1.7
N$85
  Top 0.813: R8.2 90,45.39 LAYER1.8
N$86
  Top 0.813: R9.2 94.5,45.11 LAYER2.1
N$87
  Top 0.813: R10.2 97,45.15 LAYER2.2
N$88
  Top 0.813: R11.2 99.5,45.19 LAYER2.3
N$89
  Top 0.813: R12.2 102,45.23 LAYER2.4
N$90
  Top 0.813: R13.2 104.5,45.27 LAYER2.5
N$91
  Top 0.813: R14.2 107,45.31 LAYER2.6
N$92
  Top 0.813: R15.2 109.5,45.35 LAYER2.7
N$93
  Top 0.813: R16.2 112,45.39 LAYER2.8
N$94
  Top 0.813: R17.2 116.5,45.11 LAYER3.1
N$95
  Top 0.813: R18.2 119,45.15 LAYER3.2
N$96
  Top 0.813: R19.2 121.5,45.19 LAYER3.3
N$97
  Top 0.813: R20.2 124,45.23 LAYER3.4
N$98
  Top 0.813: R21.2 126.5,45.27 LAYER3.5
N$99
  Top 0.813: R22.2 129,45.31 LAYER3.6
N$100
  Top 0.813: R23.2 131.5,45.35 LAYER3.7
N$101
  Top 0.813: R24.2 134,45.39 LAYER3.8
N$102
  Top 0.813: R25.2 138.5,45.11 LAYER4.1
N$103
  Top 0.813: R26.2 141,45.15 LAYER4.2
N$104
  Top 0.813: R27.2 143.5,45.19 LAYER4.3
N$105
  Top 0.813: R28.2 146,45.23 LAYER4.4
N$106
  Top 0.813: R29.2 148.5,45.27 LAYER4.5
N$107
  Top 0.813: R30.2 151,45.31 LAYER4.6
N$108
  Top 0.813: R31.2 153.5,45.35 LAYER4.7
N$109
  Top 0.813: R32.2 156,45.39 LAYER4.8
N$110
  Top 0.813: R33.2 72.5,18.11 LAYER5.1
N$111
  Top 0.813: R34.2 75,18.15 LAYER5.2
N$112
  Top 0.813: R35.2 77.5,18.19 LAYER5.3
N$113
  Top 0.813: R36.2 80,18.23 LAYER5.4
N$114
  Top 0.813: R37.2 82.5,18.27 LAYER5.5
N$115
  Top 0.813: R38.2 85,18.31 LAYER5.6
N$116
  Top 0.813: R39.2 87.5,18.35 LAYER5.7
N$117
  Top 0.813: R40.2 90,18.39 LAYER5.8
N$118
  Top 0.813: R41.2 94.5,18.11 LAYER6.1
N$119  (via drill 0.6)
  Top 0.406: IC11.2 45.66,38.16 47.1,39.6 v47.3,39.6
  Bottom 0.406: JP2.9 14.52,47.08 21.4,40.2 46.7,40.2 v47.3,39.6
N$120
  Top 0.813: R42.2 97,18.15 LAYER6.2
N$121
  Top 0.813: R43.2 99.5,18.19 LAYER6.3
N$122
  Top 0.813: R44.2 102,18.23 LAYER6.4
N$123
  Top 0.813: R45.2 104.5,18.27 LAYER6.5
N$124
  Top 0.813: R46.2 107,18.31 LAYER6.6
N$125
  Top 0.813: R47.2 109.5,18.35 LAYER6.7
N$126
  Top 0.813: R48.2 112,18.39 LAYER6.8
N$127
  Top 0.813: R49.2 116.5,18.11 LAYER7.1
N$128
  Top 0.813: R50.2 119,18.15 LAYER7.2
N$129
  Top 0.813: R51.2 121.5,18.19 LAYER7.3
N$130
  Top 0.813: R52.2 124,18.23 LAYER7.4
N$131
  Top 0.813: R53.2 126.5,18.27 LAYER7.5
N$132
  Top 0.813: R54.2 129,18.31 LAYER7.6
N$133
  Top 0.813: R55.2 131.5,18.35 LAYER7.7
N$134
  Top 0.813: R56.2 134,18.39 LAYER7.8
N$135
  Top 0.813: R57.2 138.5,18.11 LAYER8.1
N$136
  Top 0.813: R59.2 141,18.15 LAYER8.2
N$137
  Top 0.813: R60.2 143.5,18.19 LAYER8.3
N$138
  Top 0.813: R61.2 146,18.23 LAYER8.4
N$139
  Top 0.813: R62.2 148.5,18.27 LAYER8.5
N$140
  Top 0.813: R63.2 151,18.31 LAYER8.6
N$141
  Top 0.813: R64.2 153.5,18.35 LAYER8.7
N$142
  Top 0.813: R65.2 156,18.39 LAYER8.8
N$143  (via drill 0.6)
  Top 0.61: LAYERS.8 122.89,75.11 v130,68
  Bottom 0.61: v130,68 U$1.2
N$144
  Bottom 0.813: 120.35,69.65 LAYERS.7
  Bottom 1.016: U$2.2 120.35,69.65
N$145
  Bottom 0.813: U$3.2 113,68 117.81,72.81 LAYERS.6
N$146
  Bottom 0.813: U$4.2 129.5,76 127,78.5 117,78.5 115.27,76.77 LAYERS.5
N$147  (via drill 0.6)
  Top 0.406: IC2.14 78.95,63.45 73.5,58 v73.5,55.3 | IC11.1 44.34,38 v42,38 | JP2.1 14.89,31.3 v31.3,31.3
  Bottom 0.406: v31.3,31.3 32.3,31.3 39,38 v42,38 44.8,38 46,36.8 53.8,36.8 72.3,55.3 v73.5,55.3
N$148  (via drill 0.6)
  Top 0.61: LAYERS.4 112.73,73.73 107.5,68.5 98.1,68.5 v98,68.6
  Bottom 0.61: U$5.2 93.5,68.5 97.9,68.5 v98,68.6
N$149
  Bottom 0.813: LAYERS.3 110.19,76.81 109,78 100.5,78 99,76.5 U$6.2
N$150  (via drill 0.6)
  Top 0.61: LAYERS.2 107.65,73.65 105.8,71.8 87.8,71.8 84,68 v82.3,68
  Bottom 0.61: U$7.2 v82.3,68
N$151  (via drill 0.6)
  Top 0.61: v83.5,76.5 104.11,76.5 LAYERS.1
  Bottom 0.61: U$8.2 v83.5,76.5
N$152  (via drill 0.6)
  Top 0.406: v52,42.5 52.24,42.5 IC11.30 | v44,46.4 42.8,47.6 42.8,53.3 69,79.5 134.8,79.5 v144,70.3
  Bottom 0.406: v52,42.5 48.5,42.5 44.6,46.4 v44,46.4 | v144,70.3 U$1.1
N$153  (via drill 0.6)
  Top 0.406: IC11.31 53.11,44.5 v52,44.5 | v44.5,48.5 44.5,53.6 69.4,78.5 124,78.5 v127.5,75
  Bottom 0.406: U$2.1 128.65,73.85 v127.5,75 | v44.5,48.5 48,48.5 v52,44.5
N$154  (via drill 0.6)
  Top 0.406: IC11.32 74.47,67 85,67 88.2,70.2 100.2,70.2 v100.25,70.15
  Bottom 0.406: U$3.1 102.3,65.7 101.5,66.5 101.5,68.5 v100.25,70.15
N$155  (via drill 0.6)
  Top 0.406: IC11.33 53.27,48.27 v55,50
  Bottom 0.406: U$4.1 144.7,78.3 145.7,77.3 145.7,66.9 148.1,64.5 150.7,64.5 152.9,62.3 152.9,59.6 150,56.7 70.2,56.7 63.5,50 v55,50
N$156  (via drill 0.6)
  Top 0.406: IC11.34 50.73,48.63 72.6,70.5 v83.1,70.5
  Bottom 0.406: v83.1,70.5 83.1,69.6 85.1,67.6 85.1,66.3 85.7,65.7 U$5.1
N$157  (via drill 0.6)
  Top 0.406: IC11.35 49,47.52 49,50 72.5,73.5 v83.5,73.5
  Bottom 0.406: U$6.1 84.2,74.2 v83.5,73.5
N$158  (via drill 0.6)
  Top 0.406: IC11.36 47.5,47.89 47.5,51.2 v66.9,70.6
  Bottom 0.406: U$7.1 66.9,70.15 v66.9,70.6
N$159  (via drill 0.6)
  Top 0.406: IC11.37 46.2,48.06 46.2,52.7 v67.5,74
  Bottom 0.406: U$8.1 67.7,74.2 v67.5,74
N$160  (via drill 0.6)
  Top 0.406: v57,30.5 57,31.61 IC11.14
  Bottom 0.406: BUZZER.+ 21.1,20.5 55.5,20.5 57,22 v57,30.5
N$161  (via drill 0.6)
  Top 0.406: v63.3,41.5 63.3,42.1 60.8,44.6 58.86,44.6 IC11.26
  Bottom 0.406: START.4 55.74,10.24 63.3,17.8 v63.3,41.5
  Bottom 1.016: START.3 START.4
N$162  (via drill 0.6)
  Top 0.406: R67.2 60,18.5 61.5,20 v61.5,23.5 | v61.6,39.8 61.6,42.65 60.5,43.75 59.14,43.75 IC11.25
  Bottom 0.406: v61.5,23.5 61.6,23.6 v61.6,39.8
N$163
  Top 1.016: LED_START.A R67.1
N$164
  Top 0.406: R69.2 62.5,36.5 60.5,38.5 60.5,42.25 60,42.75 59.28,42.75 IC11.24
N$165
  Top 1.016: R69.1 65.73,37.17 STATUS_LED.2
N$166  (via drill 0.6)
  Top 0.406: IC6.10 84.67,39.92 86,41.25 104.5,41.25 105.67,40.08 | 105.67,40.08 IC7.10 105.67,39.67 | IC9.10 149.68,38.92 150,39.25 arc-7 152.25,41.25 | 152.25,41.25 129,41.25 127.67,39.92 IC8.10 127.67,40.08 126.5,41.25 106.85,41.25 105.67,40.08 | 152.25,41.25 158,41.25 | 158,41.25 159.25,42.5 159.25,59.75 152,67 150.75,67 149.94,66.19 IC5.10 149.94,62.44 v149.75,62 | IC4.10 129.13,63.37 v130.5,61.75 | v107,61.75 105.83,62.91 IC3.10 | IC2.10 84.03,62.22 v84.5,61.75 | R70.1 155.5,38.75 158,41.25
  Bottom 0.406: v149.75,62 149.5,61.75 v130.5,61.75 v107,61.75 v84.5,61.75
N$173  (via drill 6)
  other vias: 157,77
N$174  (via drill 6)
  other vias: 157,7
N$175  (via drill 6)
  other vias: 7,7
N$176  (via drill 6)
  other vias: 7,77
N$182
  Top 0.406: IC11.29 59.28,48.41 C0013.1
N$186
  Top 0.813: R58.1 POWER.A
N$187
  Top 0.406: IC11.8 45.71,31.44 KWARC.1 45.71,28.71 C101.2
N$188
  Top 0.406: IC11.7 45.34,32.21 KWARC.2 41.71,32.21 C100.2

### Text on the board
Top: Tomasz Sikorski praca inzynierska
